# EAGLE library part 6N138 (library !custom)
Optocoupler used in Arduinoboy.
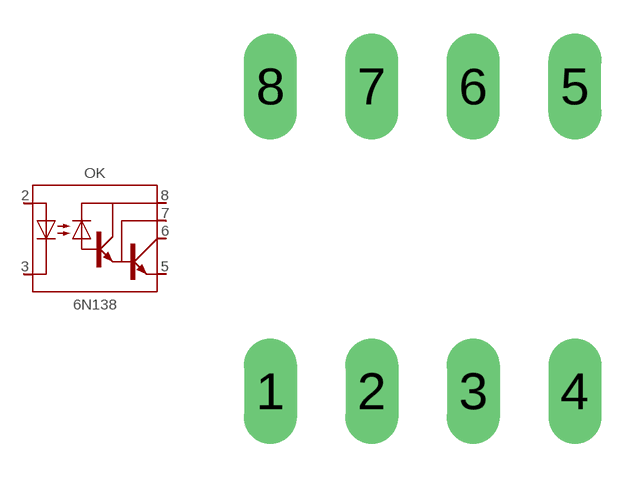
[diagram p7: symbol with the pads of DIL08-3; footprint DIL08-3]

Designator prefix OK

## 6N138  [DIL08-3]
2  A  pas
3  C  pas
5  GND  pas
6  VO  pas
7  VB  pas
8  VCC  pas

## Footprint DIL08-3 (pad centres in mm)
Dual In Line Package
drill 0.813 long: 1 -3.81,-3.81; 2 -1.27,-3.81; 3 1.27,-3.81; 4 3.81,-3.81; 5 3.81,3.81; 6 1.27,3.81; 7 -1.27,3.81; 8 -3.81,3.81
